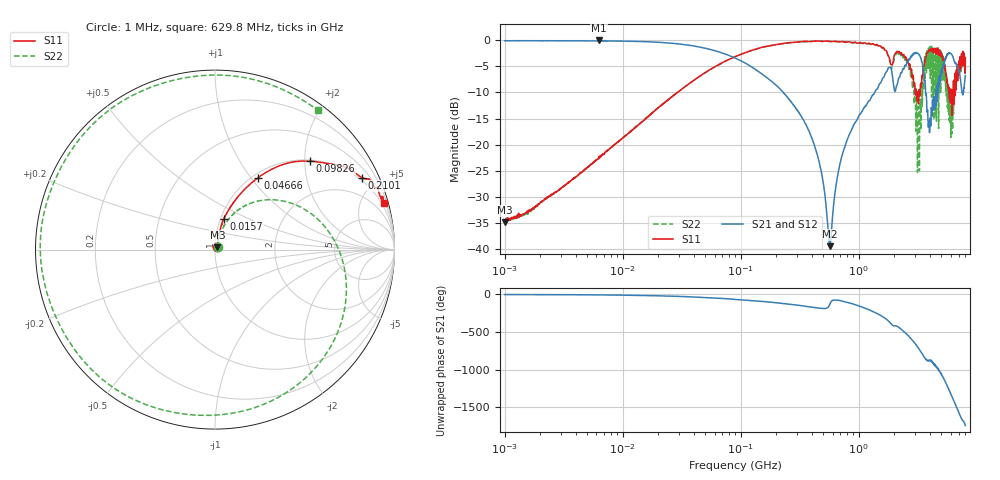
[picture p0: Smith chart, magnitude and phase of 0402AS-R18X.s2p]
!s-Parameter Generated by FASTRON Sdn. Bhd.
!FASTRON P/N : 0402AS-R18X
!Keysight Technologies: E5071C_MY46733604_B.14.02
!Date: Mon Dec 01 10:49:48 2025
!Version  :Rev00  Mon Dec 01 10:49:48 2025
!Data & Calibration Information:
!Freq  S11:SOLT2(ON)  S21:SOLT2(ON)  S12:SOLT2(ON)  S22:SOLT2(ON)
!PortZ  Port1:50+j0  Port2:50+j0
!When reading reference impedance value at option line is always used.
! Remarks : This data is being provided solely for informational purposes.
# Hz S dB R 50
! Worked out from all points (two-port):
!   1601 points, 1 MHz to 8 GHz, reference 50 ohm
!   highest |S21| = -0.08 dB at 6.301 MHz (marker M1); lowest = -39.4 dB at 569.9 MHz (marker M2)
!   |S21| within 3 dB of the highest: 2.817 GHz to 3.293 GHz (476.1 MHz wide, 15.6 % of centre); 5.525 GHz to 6.231 GHz (705.5 MHz wide, 12 % of centre)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
!   lowest |S11| = -34.8 dB at 1 MHz (marker M3), VSWR 1.04, Z = 51.4 + j1.24 ohm
!   |S11| at or under -10 dB: 3.083 GHz to 3.156 GHz (73.62 MHz wide, 2.36 % of centre); 3.164 GHz to 3.236 GHz (71.35 MHz wide, 2.23 % of centre); 5.856 GHz to 5.945 GHz (89.03 MHz wide, 1.51 % of centre)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
!   |S22| runs from -34.8 to -0.2 dB; largest |S21 - S12| = 0.016
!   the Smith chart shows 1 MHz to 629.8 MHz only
!   S11 on the Smith chart (normalised r, x): 1 MHz: 1.03, +0.02; 15.7 MHz: 1.04, +0.37; 46.66 MHz: 1.06, +1.08; 98.26 MHz: 1.03, +2.13; 210.1 MHz: 0.87, +4.16; 629.8 MHz: 0.64, +7.29
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1000000  -34.80 41.4  -0.13 -0.9  -0.13 -0.9  -34.40 40.3
4479405  -25.30 71.7  -0.15 -4.1  -0.14 -4.1  -25.30 70.1
6301378  -22.30 76.1  -0.08 -6.5  -0.19 -6.0  -22.40 70.7
1.569966e7  -15.00 74.2  -0.31 -14.0  -0.32 -13.9  -15.00 66.3
2.00676e7  -12.90 71.4  -0.42 -17.7  -0.42 -17.6  -12.90 62.5
4.665652e7  -6.65 59.1  -1.42 -38.0  -1.41 -37.9  -6.70 36.0
8.994653e7  -3.17 45.3  -3.45 -64.1  -3.44 -64.1  -3.17 -1.1
9.825861e7  -2.81 42.9  -3.86 -68.4  -3.84 -68.4  -2.80 -7.3
2.100621e8  -0.79 26.0  -9.10 -114.0  -9.09 -114.0  -0.80 -79.8
4.006501e8  -0.28 17.2  -18.80 -169.0  -18.80 -169.0  -0.22 174.0
5.698649e8  -0.28 15.7  -39.40 -125.0  -39.40 -126.0  -0.24 86.4
6.29833e8  -0.20 15.5  -29.10 -73.5  -29.10 -73.6  -0.31 53.6
9.011973e8  -0.45 15.0  -16.30 -128.0  -16.40 -128.0  -0.52 -82.8
1.080879e9  -0.65 17.7  -13.40 -170.0  -13.40 -171.0  -0.61 -172.0
1.264475e9  -0.81 22.4  -11.20 147.0  -11.20 147.0  -0.73 97.4
1.473292e9  -1.13 25.3  -8.74 96.7  -8.75 96.6  -1.11 -4.7
1.7949e9  -3.11 27.2  -5.22 3.9  -5.24 3.9  -3.49 -172.0
2.178389e9  -2.24 45.5  -7.27 -76.7  -7.27 -76.7  -2.76 8.6
2.530914e9  -3.73 42.0  -4.60 -162.0  -4.58 -162.0  -3.59 -166.0
3.203473e9  -12.20 94.9  -2.70 7.4  -2.69 7.1  -12.70 -101.0
5.752228e9  -8.68 166.0  -2.47 -171.0  -2.47 -172.0  -11.70 73.1
8e9  -3.38 -99.2  -6.84 60.1  -6.88 59.7  -6.13 127.0
